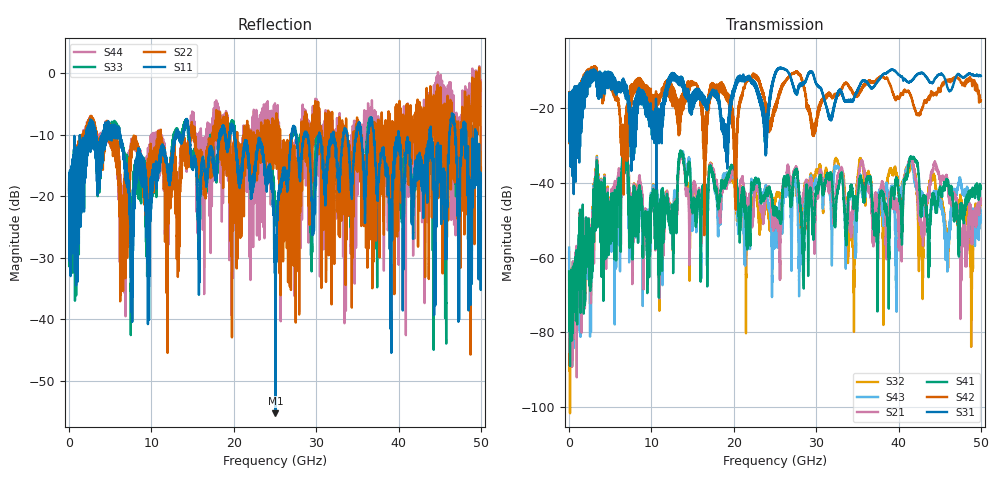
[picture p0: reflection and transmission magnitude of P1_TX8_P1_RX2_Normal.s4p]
!Keysight Technologies,N5225B,MY57041031,A.13.20.10
!Date: Friday, May 31, 2019 11:16:10
!Correction: S11(Full 4 Port(1,2,3,4))
!S12(Full 4 Port(1,2,3,4))
!S13(Full 4 Port(1,2,3,4))
!S14(Full 4 Port(1,2,3,4))
!S21(Full 4 Port(1,2,3,4))
!S22(Full 4 Port(1,2,3,4))
!S23(Full 4 Port(1,2,3,4))
!S24(Full 4 Port(1,2,3,4))
!S31(Full 4 Port(1,2,3,4))
!S32(Full 4 Port(1,2,3,4))
!S33(Full 4 Port(1,2,3,4))
!S34(Full 4 Port(1,2,3,4))
!S41(Full 4 Port(1,2,3,4))
!S42(Full 4 Port(1,2,3,4))
!S43(Full 4 Port(1,2,3,4))
!S44(Full 4 Port(1,2,3,4))
!S4P File: Measurements: <S11,S12,S13,S14>,
!<S21,S22,S23,S24>,
!<S31,S32,S33,S34>,
!<S41,S42,S43,S44>:
# Hz S  dB  R 50.0
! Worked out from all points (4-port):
!   5000 points, 10 MHz to 50 GHz, reference 50 ohm
!   strongest paths, dB at 10 MHz, 12.51 GHz, 25.01 GHz, 37.51 GHz, 50 GHz:
!     S31: -19.6, -10.8, -11.0, -12.7, -11.3
!     S42: -19.5, -16.3, -19.5, -12.4, -17.9
!     S41: -63.7, -48.3, -47.5, -55.3, -41.2
!     S21: -68.6, -48.7, -49.7, -58.7, -44.2
!     S43: -57.3, -47.9, -54.6, -43.1, -49.8
!     S32: -58.5, -50.4, -45.1, -54.5, -44.7
!   lowest |S11| = -55.3 dB at 25.05 GHz (marker M1), VSWR 1.00, Z = 49.8 + j0.0435 ohm
!   |S11| at or under -10 dB: 6.192 GHz to 12.89 GHz (6.696 GHz wide, 70.2 % of centre); 20.1 GHz to 26.99 GHz (6.893 GHz wide, 29.3 % of centre); 40 GHz to 43.77 GHz (3.765 GHz wide, 8.99 % of centre)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
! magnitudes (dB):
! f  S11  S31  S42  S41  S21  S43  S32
! 10 MHz  -19.5  -19.6  -19.5  -63.7  -68.6  -57.3  -58.5
! 6.83 GHz  -14.5  -13.8  -22.7  -30.4  -30.8  -28.9  -28.9
! 9.26 GHz  -15.7  -17.0  -17.6  -49.1  -46.8  -51.8  -48.1
! 13.64 GHz  -11.0  -12.6  -16.6  -31.6  -32.5  -31.6  -32.5
! 25.05 GHz  -55.3  -10.5  -19.6  -47.5  -51.4  -57.3  -44.9
! 27.29 GHz  -8.5  -14.5  -10.7  -38.0  -37.1  -39.3  -39.2
! 50 GHz  -22.7  -11.3  -17.9  -41.2  -44.2  -49.8  -44.7
